{attribute 'no_check'}
//Provides all information of PlcTaskSystemInfo corresponding to the caller task of the instance 
FUNCTION_BLOCK TaskInfo
VAR_INPUT
END_VAR
VAR_OUTPUT
	Index													:	INT := 0;
	TaskName          										: 	STRING(63);
	ObjId             										: 	OTCID;
	CycleTime         										: 	UDINT;
	CycleTimeT       										: 	TIME;
	CycleTimeLT       										: 	LTIME;
	CycleTimeFloat											:	LREAL;	
	Priority          										: 	UINT;
	AdsPort           										: 	UINT;
	CycleCount        										: 	UDINT;
	Tasktime												:	ULINT;
	DcTaskTime        										: 	T_DCTIME64;
	LastExecTime      										: 	UDINT; 
	LastExecTimeNS      									: 	UDINT; //Converted in ns 
	LastExecTimeLT      									: 	LTIME; 
	MaxExecTimeLT											:	LTIME;
	FirstCycle        										: 	BOOL;
	CycleTimeExceeded 										: 	BOOL;	
	CycleTimeExceededCount 									: 	UDINT; //Set to 0 via method resetCylceTimeExceeded()
	CycleTimeExceededCountTotal 							: 	UDINT; //Overall count cycle time exeeded
	InCallAfterOutputUpdate									:	BOOL;
	RTViolation												:	BOOL;
END_VAR

VAR
	GETCURTASKINDEX											: 	GETCURTASKINDEX;
	GETTASKTIME												:	GETTASKTIME;
	TaskInterlock											:	BOOL;
END_VAR

	(*	evaluate PlcTaskInfo arrays													*)
	(********************************************************************************)

(* read task info array of caller task ************************************************************************)
	IF GETCURTASKINDEX.index = 0 	
	THEN 
		GETCURTASKINDEX(index => index); 
		//Init
		TaskName          									:= TwinCAT_SystemInfoVarList._TaskInfo[index].TaskName;
		ObjId             									:= TwinCAT_SystemInfoVarList._TaskInfo[index].ObjId;
		CycleTime         									:= TwinCAT_SystemInfoVarList._TaskInfo[index].CycleTime;
		Priority          									:= TwinCAT_SystemInfoVarList._TaskInfo[index].Priority;
		AdsPort           									:= TwinCAT_SystemInfoVarList._TaskInfo[index].AdsPort;
		CycleTimeT											:= LREAL_TO_TIME(UDINT_TO_LREAL(CycleTime) * 0.0001 );
		CycleTimeLT											:= TO_LTIME(CycleTime * 100);
		CycleTimeFloat										:= (UDINT_TO_LREAL(CycleTime) * 0.0001 / 1000.0);		
	END_IF

	//Cylic 
	CycleCount        										:= TwinCAT_SystemInfoVarList._TaskInfo[index].CycleCount;
	DcTaskTime        										:= TO_ULINT(TwinCAT_SystemInfoVarList._TaskInfo[index].DcTaskTime); 
	LastExecTime      										:= TwinCAT_SystemInfoVarList._TaskInfo[index].LastExecTime; 
	LastExecTimeNS											:= TwinCAT_SystemInfoVarList._TaskInfo[index].LastExecTime * 100;
	LastExecTimeLT      									:= TO_LTIME(LastExecTimeNS); //Converted into ns 
	MaxExecTimeLT											:= MAX(LastExecTimeLT,MaxExecTimeLT);
	
	FirstCycle        										:= TwinCAT_SystemInfoVarList._TaskInfo[index].FirstCycle;
	CycleTimeExceeded 										:= TwinCAT_SystemInfoVarList._TaskInfo[index].CycleTimeExceeded;
	IF CycleTimeExceeded 
	THEN
		CycleTimeExceededCount								:= CycleTimeExceededCount + 1;	
		CycleTimeExceededCountTotal							:= CycleTimeExceededCountTotal + 1;
	END_IF
	InCallAfterOutputUpdate									:= TwinCAT_SystemInfoVarList._TaskInfo[index].InCallAfterOutputUpdate;
	RTViolation												:= TwinCAT_SystemInfoVarList._TaskInfo[index].RTViolation;
	
	//Read time when task suppose to start
	GETTASKTIME(timeLoDW => Tasktime);	
	MEMCPY(ADR(Tasktime) + SIZEOF(GETTASKTIME.timeHiDW),ADR(GETTASKTIME.timeHiDW),SIZEOF(GETTASKTIME.timeHiDW));
	
(**************************************************************************************************)

METHOD PUBLIC resetCylceTimeExceeded : BOOL //Return value = TRUE if execution finished
VAR_INPUT
END_VAR
IF TestAndSet(TaskInterlock)
THEN
	CycleTimeExceededCount									:= 0;
	TaskInterlock											:= FALSE;
	resetCylceTimeExceeded											:= TRUE;
END_IF
END_METHOD

END_FUNCTION_BLOCK
